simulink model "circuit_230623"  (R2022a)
settings: Solver=VariableStepAuto  StartTime=0.0  StopTime=1e-4  RelTol=1e-3  AbsTol=1e-3
libraries: fl_lib x9, nesl_utility x4, ee_lib x1

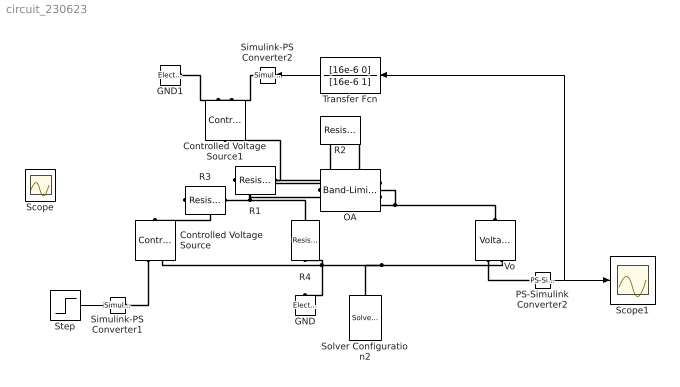
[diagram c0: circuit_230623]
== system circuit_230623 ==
  Controlled Voltage Source : fl_lib/Electrical/Electrical Sources/Controlled Voltage Source
  Controlled Voltage Source1 : fl_lib/Electrical/Electrical Sources/Controlled Voltage Source
  GND : fl_lib/Electrical/Electrical Elements/Electrical Reference
  GND1 : fl_lib/Electrical/Electrical Elements/Electrical Reference
  OA : ee_lib/Integrated Circuits/Band-Limited Op-Amp  A=2e5  Rin=1e8 Ohm  Rout=0 Ohm  Vmin=-15 V  Vmax=15 V  Vdotmax=1e7 V/s  f=5 Hz  V0=0 V
  PS-Simulink Converter2 : nesl_utility/PS-Simulink Converter  PhysicalDomain=network_engine_domain  SubClassName=ps_output  LeftPortType=input  RightPortType=output  PseudoPeriodic=off  Frequencies=[]  VectorFormat=1-D array  Unit=inherit  AffineConversion=off
  R1 : fl_lib/Electrical/Electrical Elements/Resistor  R=10 kOhm  i_specify=off  i_priority=None  i=0 A  i_nominal_specify=off  i_nominal_unit=A  i_nominal_value=1  v_specify=off  v_priority=None  v=0 V  v_nominal_specify=off  v_nominal_unit=V  v_nominal_value=1
  R2 : fl_lib/Electrical/Electrical Elements/Resistor  R=10 MOhm  i_specify=off  i_priority=None  i=0 A  i_nominal_specify=off  i_nominal_unit=A  i_nominal_value=1  v_specify=off  v_priority=None  v=0 V  v_nominal_specify=off  v_nominal_unit=V  v_nominal_value=1
  R3 : fl_lib/Electrical/Electrical Elements/Resistor  R=10 kOhm  i_specify=off  i_priority=None  i=0 A  i_nominal_specify=off  i_nominal_unit=A  i_nominal_value=1  v_specify=off  v_priority=None  v=0 V  v_nominal_specify=off  v_nominal_unit=V  v_nominal_value=1
  R4 : fl_lib/Electrical/Electrical Elements/Resistor  R=10 MOhm  i_specify=off  i_priority=None  i=0 A  i_nominal_specify=off  i_nominal_unit=A  i_nominal_value=1  v_specify=off  v_priority=None  v=0 V  v_nominal_specify=off  v_nominal_unit=V  v_nominal_value=1
  Scope1 : Scope
  Simulink-PS Converter1 : nesl_utility/Simulink-PS Converter  PhysicalDomain=network_engine_domain  SubClassName=ps_input  LeftPortType=input  RightPortType=output  PseudoPeriodic=off  Frequencies=[]  NoiseDistribution=none  NoiseParameters=[]  Unit=1  AffineConversion=off  FilteringAndDerivatives=provide  SimscapeFilterOrder=1  InputFilterTimeConstant=0.001  UdotUserProvided=0
  Simulink-PS Converter2 : nesl_utility/Simulink-PS Converter  PhysicalDomain=network_engine_domain  SubClassName=ps_input  LeftPortType=input  RightPortType=output  PseudoPeriodic=off  Frequencies=[]  NoiseDistribution=none  NoiseParameters=[]  Unit=1  AffineConversion=off  FilteringAndDerivatives=provide  SimscapeFilterOrder=1  InputFilterTimeConstant=0.001  UdotUserProvided=0
  Solver Configuration2 : nesl_utility/Solver Configuration  PhysicalDomain=network_engine_domain  SubClassName=solver  LeftPortType=input  RightPortType=generic  Tones=[]  Harmonics=[]  SimulateNoise=off  Profile=off  UseLocalSampling=off  EnableSwitchedLinearOptims=on  FrequencyDomain=off  UseCCode=off  RelTol=0.001  AbsTol=1e-06  MinStep=1e-09  ToWorkspace=off  RevertToSquareIcSolve=off  NumHomotopyIterations=100  PhasorMode=off  PhasorModeNumHarmonics=1  IndexReductionMethod=DerivativeReplacement  DoDC=off  ResidualTolerance=1e-09  UseLocalSolver=off  LocalSolverChoice=NE_BACKWARD_EULER_ADVANCER  LocalSolverSampleTime=0.001  DoFixedCost=off  MaxNonlinIter=3  MaxModeIter=2  ComputeImpulses=off  ImpulseIterations=2  LinearAlgebra=Sparse  LinearAlgebraNumThread=0  EquationFormulation=NE_TIME_EF  DelaysMemoryBudget=1024  AutomaticFiltering=off  FilteringTimeConstant=0.001  PartitionStorageMethod=AS_NEEDED  PartitionMemoryBudget=1024  PartitionMethod=FAST
  Step : Step  Time=0  SampleTime=0
  Transfer Fcn : TransferFcn  Numerator=[16e-6 0]  Denominator=[16e-6 1]
  Vo : fl_lib/Electrical/Electrical Sensors/Voltage Sensor
  Scope : Scope
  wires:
  Step/1 -> Simulink-PS Converter1/1
  PS-Simulink Converter2/1 -> Transfer Fcn/1, Scope1/1
  Transfer Fcn/1 -> Simulink-PS Converter2/1
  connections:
  Vo/LConn1 -- R2/LConn1 -- OA/RConn1
  Controlled Voltage Source/RConn1 -- Simulink-PS Converter1/RConn1
  R1/LConn1 -- R2/RConn1 -- OA/LConn2
  R3/RConn1 -- Controlled Voltage Source/LConn1
  R3/LConn1 -- R4/RConn1 -- OA/LConn1
  Vo/RConn2 -- Solver Configuration2/RConn1 -- R4/LConn1 -- Controlled Voltage Source/RConn2 -- GND/LConn1
  R1/RConn1 -- Controlled Voltage Source1/LConn1
  Vo/RConn1 -- PS-Simulink Converter2/LConn1
  Simulink-PS Converter2/RConn1 -- Controlled Voltage Source1/RConn1
  GND1/LConn1 -- Controlled Voltage Source1/RConn2
